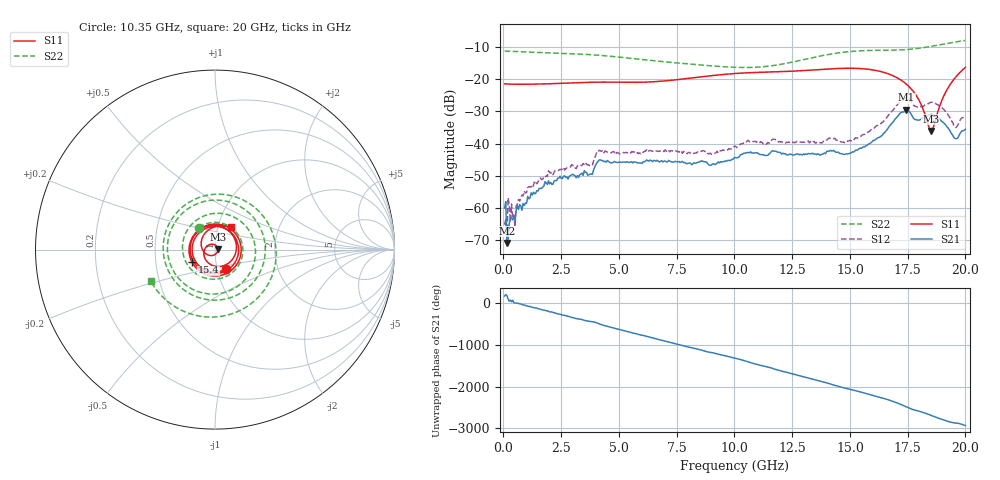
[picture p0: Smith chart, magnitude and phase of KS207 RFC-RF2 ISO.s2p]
!Agilent	"Technologies,E8364B,MY43040668,A.07.50.67"
!Agilent	E8364B:	A.07.50.67
!Date:	"Friday,"	June	"03,"	2022	13:37:20
!Correction:	S11(Full	2	"Port(1,2))"
!S21(Full	2	"Port(1,2))"
!S12(Full	2	"Port(1,2))"
!S22(Full	2	"Port(1,2))"
!S2P	File:	Measurements:	"S11,"	"S21,"	"S12,"	S22:
#	Hz	S	dB	R	50
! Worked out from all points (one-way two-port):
!   400 points, 50 MHz to 20 GHz, reference 50 ohm
!   highest |S21| = -29.53 dB at 17.45 GHz (marker M1); lowest = -70.9 dB at 150 MHz (marker M2)
!   lowest |S11| = -36.1 dB at 18.5 GHz (marker M3), VSWR 1.03, Z = 51.6 + j0.309 ohm
!   |S11| at or under -10 dB: start of sweep to end of sweep
!   |S22| runs from -16.4 to -8.0 dB; largest |S21 - S12| = 0.019
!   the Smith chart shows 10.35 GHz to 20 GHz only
!   S11 on the Smith chart (normalised r, x): 10.35 GHz: 1.10, -0.24; 15.4 GHz: 0.77, -0.11; 20 GHz: 1.15, +0.29
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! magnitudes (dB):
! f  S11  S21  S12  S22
! 50 MHz  -21.5  -60.0  -65.3  -11.3
! 100 MHz  -21.5  -58.1  -63.6  -11.3
! 150 MHz  -21.5  -70.9  -71.9  -11.3
! 200 MHz  -21.5  -69.8  -56.9  -11.3
! 300 MHz  -21.5  -63.4  -64.3  -11.3
! 350 MHz  -21.6  -63.1  -58.8  -11.4
! 500 MHz  -21.6  -64.0  -65.9  -11.4
! 550 MHz  -21.6  -60.8  -59.4  -11.4
! 650 MHz  -21.6  -60.5  -57.4  -11.5
! 1.35 GHz  -21.6  -55.6  -51.6  -11.7
! 3.4 GHz  -21.1  -49.2  -46.8  -12.2
! 4.15 GHz  -20.9  -45.1  -42.1  -12.6
! 6.7 GHz  -20.7  -45.4  -42.5  -14.4
! 10.05 GHz  -18.2  -44.4  -40.9  -16.3
! 10.35 GHz  -18.1  -43.3  -40.2  -16.4
! 13.35 GHz  -17.2  -43.1  -39.7  -13.4
! 15.4 GHz  -16.7  -41.6  -37.9  -11.2
! 16.7 GHz  -18.4  -34.7  -31.0  -11.0
! 17.45 GHz  -21.6  -29.5  -25.7  -10.8
! 18.5 GHz  -36.1  -31.0  -27.2  -9.8
! 19.6 GHz  -19.2  -38.5  -35.0  -8.4
! 20 GHz  -16.3  -35.6  -31.4  -8.0
